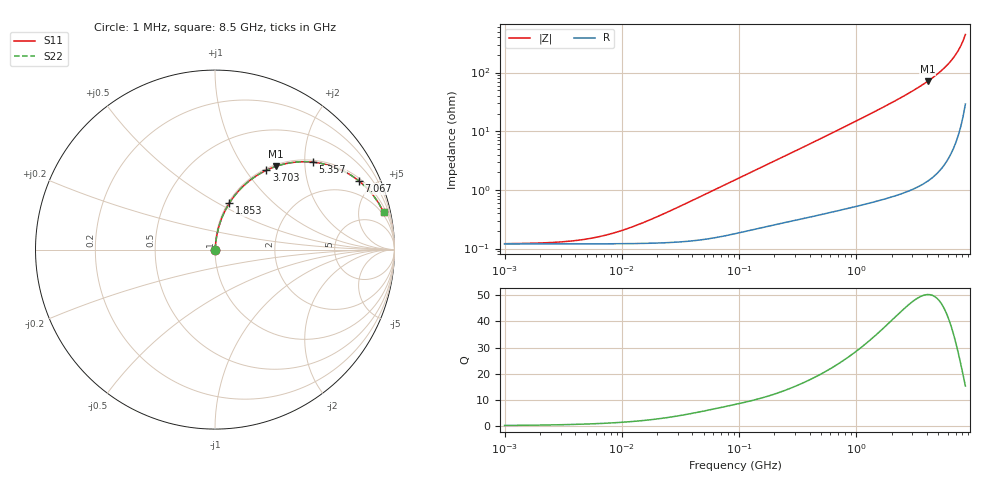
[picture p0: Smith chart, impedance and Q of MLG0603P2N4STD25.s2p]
! S-Parameter Data Generated by TDK Corporation
! Copyright(C) 2025 TDK Corporation.
! All Rights Reserved.
! TDK P/N: MLG0603P2N4STD25 (SMD / SMT Inductor (Coil))
! Property: L=2.4nH at 500MHz
! Size(LxWxT): 0.6x0.3x0.3mm
! Model Type: s2p (Touchstone File Format Version 1.0)
! Frequency: DC=Yes Start=1MHz Stop=8500MHz 198points Log-sweep
! Model Generated on Feb. 6, 2025
! Terms and conditions regarding TDK Simulation Models:
! 1)This simulation model is being provided solely for informational
!  purposes. Please refer to the specifications of the products in
!  terms of detailed characteristics of such products.
! 2)In no event shall TDK Corporation of any of its subsidiaries be
!  liable for any loss or damage arising, directly or indirectly,
!  from any information contained in this simulation model, including,
!  but not limited to loss or damages arising from any inaccuracies,
!  omissions or errors in connection with such information.
! 3)Any and all copyrights on this simulation model are owned by
!  TDK Corporation.  Duplication or redistribution of this simulation
!  model without prior written permission from TDK Corporation
!  is prohibited.
! 4)This simulation model is subject to any modification or change
!  without any prior notice.
! 5)Neither TDK Corporation nor any of its subsidiaries shall make any
!  warranty, express or implied, including but not limited to the
!  correctness, implied warranties of merchantability and fitness for
!  a particular purpose with respect to this simulation models.
! 6)The use of this simulation model shall be deemed to have consented
!  to the terms and conditions hereof.
! Port Assignments:
!  1 ---@@@--- 2
! Applicable Conditions:
!  Temperature = 25 degC
!  DC Bias Current = 0 A
!  Small Signal Operation
# Hz S MA R 50
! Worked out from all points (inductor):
!   197 points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, 1 MHz to 8.5 GHz, reference 50 ohm
!   read as one part in series: L = 2.59 nH near 24.17 MHz
!   highest Q = 50.3 at 4.061 GHz (marker M1), where L = 2.79 nH
!   S11 on the Smith chart (normalised r, x): 1 MHz: 1.00, +0.00; 1.853 GHz: 1.01, +0.57; 3.703 GHz: 1.03, +1.26; 5.357 GHz: 1.05, +2.19; 7.067 GHz: 1.13, +4.12; 8.5 GHz: 1.58, +8.90
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1000000  0.00121 7.7  0.9988 -0.0  0.9988 -0.0  0.00121 7.7
2517452  0.001268 18.9  0.9988 -0.0  0.9988 -0.0  0.001268 18.9
4587603  0.001415 31.9  0.9988 -0.0  0.9988 -0.0  0.001415 31.9
6636977  0.001619 41.9  0.9988 -0.1  0.9988 -0.1  0.001619 41.9
9168677  0.001923 51.0  0.9988 -0.1  0.9988 -0.1  0.001923 51.0
1.326451e7  0.002483 60.5  0.9988 -0.1  0.9988 -0.1  0.002483 60.5
2.10461e7  0.003648 69.9  0.9987 -0.2  0.9987 -0.2  0.003648 69.9
9.219544e7  0.01474 82.2  0.9981 -0.8  0.9981 -0.8  0.01474 82.2
4.229561e8  0.06373 83.2  0.9945 -3.6  0.9945 -3.6  0.06373 83.2
9.270694e8  0.1371 80.0  0.9856 -7.9  0.9856 -7.9  0.1371 80.0
1.852819e9  0.2702 72.9  0.9559 -15.7  0.9559 -15.7  0.2702 72.9
1.940355e9  0.2826 72.2  0.9522 -16.4  0.9522 -16.4  0.2826 72.2
2.80715e9  0.4049 64.9  0.9057 -23.9  0.9057 -23.9  0.4049 64.9
3.703002e9  0.5272 57.0  0.8393 -31.8  0.8393 -31.8  0.5272 57.0
4.061159e9  0.5743 53.8  0.8073 -35.0  0.8073 -35.0  0.5743 53.8
4.664383e9  0.6504 48.3  0.7465 -40.6  0.7465 -40.6  0.6504 48.3
5.357206e9  0.7313 41.8  0.6665 -47.0  0.6665 -47.0  0.7313 41.8
6.152938e9  0.813 34.2  0.5626 -54.4  0.5626 -54.4  0.813 34.2
7.066863e9  0.8885 25.6  0.4315 -62.6  0.4315 -62.6  0.8885 25.6
7.750377e9  0.9307 19.2  0.3289 -68.4  0.3289 -68.4  0.9307 19.2
8.116539e9  0.9481 15.9  0.2735 -71.2  0.2735 -71.2  0.9481 15.9
8.5e9  0.9625 12.4  0.2158 -73.8  0.2158 -73.8  0.9625 12.4
